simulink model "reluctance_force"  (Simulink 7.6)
settings: Solver=ode15s  StartTime=0.0  StopTime=0.2  RelTol=1e-3
StopFcn:
  | close all
  | load es.mat
  | plotyy(es(1,:),es(2,:),es(1,:),es(3,:))
  | title('Vitesse et position linéaires - Reluctance Force Actuator')
  | xlabel('temps')
  | grid
  | 
  | delete *.mat
libraries: fl_lib x13, nesl_utility x6

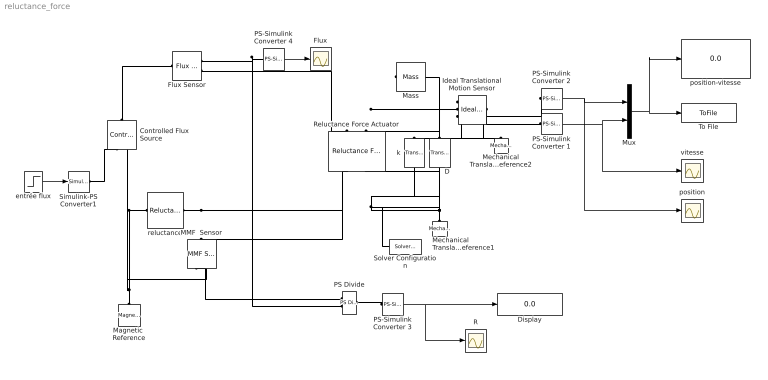
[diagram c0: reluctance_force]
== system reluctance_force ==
  Controlled Flux Source : fl_lib/Magnetic/Magnetic Sources/Controlled Flux Source  DialogController=NetworkEngine.DynNeDlgSource  SystemSampleTime=-1  phi_Log=off  mmf_Log=off  LocalVarNames=|phi|mmf  LocalVarDescs=|phi|mmf  LocalVarLogging=[0 0]
  D : fl_lib/Mechanical/Translational Elements/Translational Damper  DialogController=NetworkEngine.DynNeDlgSource  SystemSampleTime=-1  D=100 N/(m/s)  f_Log=off  v_Log=off  LocalVarNames=|force|rel_velocity|power  LocalVarDescs=|Damping force (N)|Damper relative velocity (m/s)|Power dissipated in the damper (W)  LocalVarLogging=[0 0 0]
  Display : Display
  Flux : Scope
  Flux Sensor : fl_lib/Magnetic/Magnetic Sensors/Flux Sensor  DialogController=NetworkEngine.DynNeDlgSource  SystemSampleTime=-1  phi_Log=off  mmf_Log=off  LocalVarNames=|phi|mmf  LocalVarDescs=|phi|mmf  LocalVarLogging=[0 0]
  Ideal Translational Motion Sensor : fl_lib/Mechanical/Mechanical Sensors/Ideal Translational Motion Sensor  DialogController=NetworkEngine.DynNeDlgSource  SystemSampleTime=-1  offset=0 mm  v_Log=off  f_Log=off  x_Log=off  LocalVarNames=|v|f|x  LocalVarDescs=|v|f|x  LocalVarLogging=[]
  MMF  Sensor : fl_lib/Magnetic/Magnetic Sensors/MMF Sensor  DialogController=NetworkEngine.DynNeDlgSource  SystemSampleTime=-1  phi_Log=off  mmf_Log=off  LocalVarNames=|phi|mmf  LocalVarDescs=|phi|mmf  LocalVarLogging=[0 0]
  Magnetic  Reference : fl_lib/Magnetic/Magnetic Elements/Magnetic Reference  DialogController=NetworkEngine.DynNeDlgSource  SystemSampleTime=-1  phi_Log=off  LocalVarNames=|phi  LocalVarDescs=|phi  LocalVarLogging=0
  Mass : fl_lib/Mechanical/Translational Elements/Mass  DialogController=NetworkEngine.DynNeDlgSource  SystemSampleTime=-1  mass=1 kg  initial_velocity=0 m/s  f_Log=off  LocalVarNames=|force|velocity  LocalVarDescs=|Inertia force (N)|Mass absolute velocity (m/s)  LocalVarLogging=[0 0]
  Mechanical Translational Reference1 : fl_lib/Mechanical/Translational Elements/Mechanical Translational Reference  DialogController=NetworkEngine.DynNeDlgSource  SystemSampleTime=-1  f_Log=off  LocalVarNames=|f  LocalVarDescs=|f  LocalVarLogging=[]
  Mechanical Translational Reference2 : fl_lib/Mechanical/Translational Elements/Mechanical Translational Reference  DialogController=NetworkEngine.DynNeDlgSource  SystemSampleTime=-1  f_Log=off  LocalVarNames=|f  LocalVarDescs=|f  LocalVarLogging=[]
  Mux : Mux  Inputs=2
  PS Divide : fl_lib/Physical Signals/Functions/PS Divide  DialogController=NetworkEngine.DynNeDlgSource  SystemSampleTime=-1  LocalVarLogging=[]
  PS-Simulink Converter 1 : nesl_utility/PS-Simulink Converter  DialogController=NetworkEngine.DynNeUtilDlgSource  SystemSampleTime=-1  PhysicalDomain=network_engine_domain  LeftPortType=input  RightPortType=output  SubClassName=ps_output  Unit=1  AffineConversion=off
  PS-Simulink Converter 2 : nesl_utility/PS-Simulink Converter  DialogController=NetworkEngine.DynNeUtilDlgSource  SystemSampleTime=-1  PhysicalDomain=network_engine_domain  LeftPortType=input  RightPortType=output  SubClassName=ps_output  Unit=1  AffineConversion=off
  PS-Simulink Converter 3 : nesl_utility/PS-Simulink Converter  DialogController=NetworkEngine.DynNeUtilDlgSource  SystemSampleTime=-1  PhysicalDomain=network_engine_domain  LeftPortType=input  RightPortType=output  SubClassName=ps_output  Unit=1  AffineConversion=off
  PS-Simulink Converter 4 : nesl_utility/PS-Simulink Converter  DialogController=NetworkEngine.DynNeUtilDlgSource  SystemSampleTime=-1  PhysicalDomain=network_engine_domain  LeftPortType=input  RightPortType=output  SubClassName=ps_output  Unit=Wb  AffineConversion=off
  R : Scope
  Reluctance Force Actuator : fl_lib/Magnetic/Magnetic Elements/Reluctance Force Actuator  DialogController=NetworkEngine.DynNeDlgSource  SystemSampleTime=-1  x0=5 mm  xmin=1e-9 mm  CSA=5 mm^2  mur=1  K_contact=1e6 N/m  D_contact=50 N/(m/s)  mmf_Log=off  phi_Log=off  f_Log=off  u_Log=off  x_Log=off  LocalVarNames=|mmf|phi|f|u|x  LocalVarDescs=|mmf|phi|f|u|x  LocalVarLogging=[0 0 0 0 0]
  Simulink-PS Converter1 : nesl_utility/Simulink-PS Converter  DialogController=NetworkEngine.DynNeUtilDlgSource  SystemSampleTime=-1  PhysicalDomain=network_engine_domain  LeftPortType=input  RightPortType=output  SubClassName=ps_input  Unit=1  AffineConversion=off  InputFilterTimeConstant=.001  UdotUserProvided=0
  Solver Configuration : nesl_utility/Solver Configuration  DialogController=NetworkEngine.DynNeUtilDlgSource  SystemSampleTime=-1  PhysicalDomain=network_engine_domain  LeftPortType=input  RightPortType=generic  SubClassName=solver  Accelerate=off  Profile=off  ResidualTolerance=1e-9  MaxNonlinIter=3  MaxModeIter=2  DoFixedCost=off  UseLocalSampling=off  DoDC=off  LinearAlgebra=Sparse  LocalSolverSampleTime=.001  LocalSolverChoice=NE_BACKWARD_EULER_ADVANCER  UseLocalSolver=off
  To File : ToFile  Filename=es.mat  MatrixName=es
  entrée flux : Step  Time=0.005  After=1e-5  SampleTime=0
  k : fl_lib/Mechanical/Translational Elements/Translational Spring  DialogController=NetworkEngine.DynNeDlgSource  SystemSampleTime=-1  spr_rate=200 N/m  init_def=0 mm  f_Log=off  v_Log=off  x_Log=off  LocalVarNames=|force|deformation  LocalVarDescs=|Spring force (N)|Spring deformation (m)  LocalVarLogging=[0 0]
  position : Scope
  position-vitesse : Display
  reluctance : fl_lib/Magnetic/Magnetic Elements/Reluctance  DialogController=NetworkEngine.DynNeDlgSource  SystemSampleTime=-1  g=0.7 mm  CSA=5 cm^2  mur=1  phi_Log=off  mmf_Log=off  LocalVarNames=|phi|mmf  LocalVarDescs=|phi|mmf  LocalVarLogging=[0 0]
  vitesse : Scope
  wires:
  PS-Simulink Converter 4/1 -> Flux/1
  entrée flux/1 -> Simulink-PS Converter1/1
  Mux/1 -> To File/1, position-vitesse/1
  PS-Simulink Converter 2/1 -> Mux/1, position/1
  PS-Simulink Converter 1/1 -> Mux/2, vitesse/1
  PS-Simulink Converter 3/1 -> R/1, Display/1
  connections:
  Mechanical Translational Reference1/LConn1 -- Reluctance Force Actuator/RConn2 -- Solver Configuration/RConn1 -- k/RConn1 -- D/RConn1
  Controlled Flux Source/RConn2 -- reluctance/LConn1 -- Magnetic  Reference/LConn1 -- MMF  Sensor/RConn2
  Simulink-PS Converter1/RConn1 -- Controlled Flux Source/RConn1
  Ideal Translational Motion Sensor/RConn1 -- Mechanical Translational Reference2/LConn1
  Flux Sensor/RConn2 -- Reluctance Force Actuator/LConn1
  Controlled Flux Source/LConn1 -- Flux Sensor/LConn1
  PS-Simulink Converter 2/LConn1 -- Ideal Translational Motion Sensor/RConn3
  Ideal Translational Motion Sensor/RConn2 -- PS-Simulink Converter 1/LConn1
  Reluctance Force Actuator/LConn2 -- k/LConn1 -- Mass/LConn1 -- D/LConn1 -- Ideal Translational Motion Sensor/LConn1
  PS-Simulink Converter 3/LConn1 -- PS Divide/RConn1
  PS Divide/LConn2 -- PS-Simulink Converter 4/LConn1 -- Flux Sensor/RConn1
  PS Divide/LConn1 -- MMF  Sensor/RConn1
  Reluctance Force Actuator/RConn1 -- reluctance/RConn1 -- MMF  Sensor/LConn1
